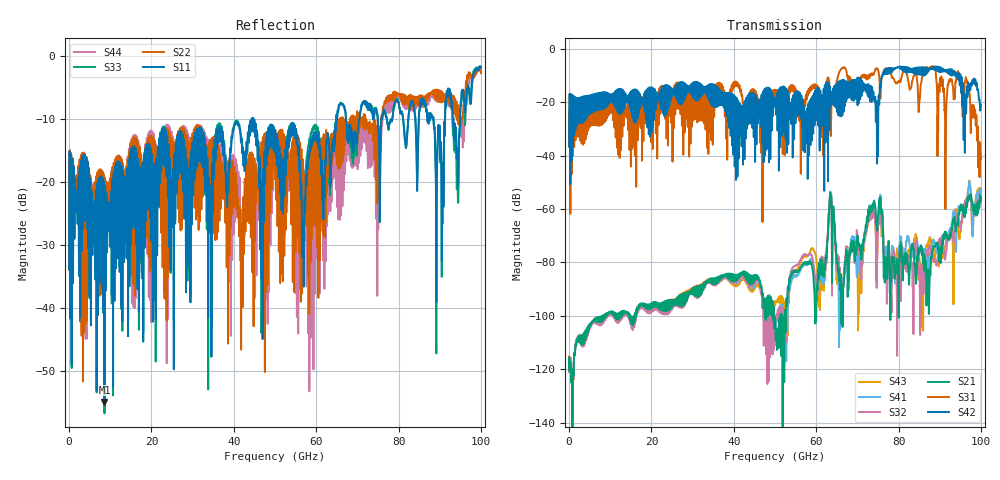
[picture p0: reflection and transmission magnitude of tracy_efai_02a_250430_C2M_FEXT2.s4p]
!! PART DESCRIPTION: TE 224G+ VSR Channel- Chip to module, IO connector to CPC(Co-packaged connector) through over the board cable
!! CHANNEL DESCRIPTION: Module trace -> Mated IO 224G+ Connector -> Internal Cable Termination -> 30AWG 300mm Cable -> Cable
!!  termination + CPC connector(No footprint or package included)
!! MODEL REVISION:  Rev 3, Created on April 29, 2025
!! MODEL STATUS: Development
!! MODEL GEOMETRY: FEXT2
!! MODEL FREQUENCY RANGE: 0 GHz to 100 GHz in 10.00 MHz frequency steps
!! PORT DEFINITIONS:
!! Port  1  ----->  Module Side  -->  Host Side  <-----  Port  2
!! Port  3  ----->  Module Side  -->  Host Side  <-----  Port  4
# HZ S MA R 45.000000
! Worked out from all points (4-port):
!   10000 points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, 10 MHz to 100 GHz, reference 45 ohm
!   strongest paths, dB at 10 MHz, 25.01 GHz, 50.01 GHz, 75.01 GHz, 100 GHz:
!     S42: -36.7, -17.8, -20.2, -37.2, -20.9
!     S31: -36.5, -17.8, -16.0, -7.7, -40.6
!     S21: -120.4, -94.2, -100.6, -62.6, -55.3
!     S32: -121.0, -94.7, -103.6, -65.3, -56.0
!     S41: -121.1, -94.6, -102.9, -61.6, -52.7
!     S43: -120.3, -93.9, -96.2, -64.6, -52.6
!   lowest |S11| = -54.9 dB at 8.6 GHz (marker M1), VSWR 1.00, Z = 44.9 + j0.15 ohm
!   |S11| at or under -10 dB: start of sweep to 44.32 GHz; 44.72 GHz to 64.9 GHz (20.18 GHz wide, 36.8 % of centre); 67.23 GHz to 70.41 GHz (3.185 GHz wide, 4.63 % of centre)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
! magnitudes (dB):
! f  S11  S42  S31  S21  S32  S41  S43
! 10 MHz  -33.8  -36.7  -36.5  -120.4  -121.0  -121.1  -120.3
! 8.6 GHz  -54.9  -22.3  -27.5  -99.7  -100.6  -100.6  -100.2
! 61.76 GHz  -25.9  -16.4  -33.2  -81.4  -78.8  -82.2  -82.3
! 63.31 GHz  -17.1  -14.1  -16.6  -55.9  -56.1  -55.8  -56.0
! 65.35 GHz  -8.7  -15.9  -10.1  -83.6  -79.0  -86.7  -86.5
! 88.17 GHz  -9.4  -7.5  -7.5  -75.5  -77.8  -72.2  -74.1
! 100 GHz  -1.8  -20.9  -40.6  -55.3  -56.0  -52.7  -52.6
